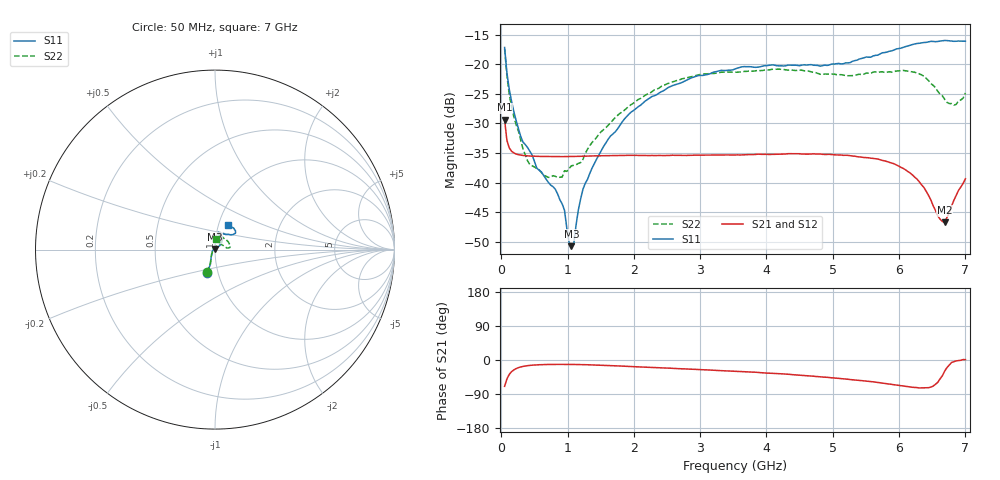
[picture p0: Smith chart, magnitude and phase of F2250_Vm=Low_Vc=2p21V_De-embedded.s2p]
! Integrated Device Technology
! Corporate Headquarters
! 6024 Silver Creek Valley Road
! San Jose, CA 95138  USA
! Phone:  1-408-284-8200
! Toll Free:  1-800-223-1366
! Webpage:  http://www.idt.com/
! Timing and RF Division
! 515 Groton Road, Suite 102
! Westford, MA 01886-6024
! Device:  F2250
! Description: Voltage Variable RF Attenuator
! Frequency:  50.0 -  6000.00 MHz
! Package:  3x3 mm Thin QFN Plastic Package: 16 pin
! Ports:  2 RF, 3 DC
!  Pin  1  = GND
!  Pin  2  = NC
!  Pin  3  = RF1  = Port 1
!  Pin  4  = NC
!  Pin  5  = GND
!  Pin  6  = GND
!  Pin  7  = GND
!  Pin  8  = GND
!  Pin  9  = NC
!  Pin 10  = RF2  = Port 2
!  Pin 11  = NC
!  Pin 12  = GND
!  Pin 13  = GND
!  Pin 14  = VCNTRL
!  Pin 15  = VDD
!  Pin 16  = VMODE
! Vcntrl:  2.210 Volts
! Vmode:  +0.000 Volts
! Vdd:  +3.30  Volts
! Current:  1.178 mA
! Data:  The device was measured on a the F2250 evaluation board which has
!  individual transmission lines to the RF pins.  Data was collected
!  using a calibrated network analyzer.  The evaluation board was
!  de-embedded using a TRL calibration technique.
!  The reference plane is the edge of the package pin.
! Misc:  SN 10
!  Action Tracker AT0258
! Date Measured:  2014-11-26
! Date:  2015-10-15  MJV
! Note:
!  Integrated Device Technology supplies this data as a sample of measured
!  data at the package pin for this product.  Your particular data for this
!  product may vary.
!  Data was taken at 25 degrees C.
!  Integrated Device Technology reserves the right to change this data at anytime.
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# GHz S dB R 50
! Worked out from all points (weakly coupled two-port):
!   201 points, 50 MHz to 7 GHz, reference 50 ohm
!   highest |S21| = -29.38 dB at 50 MHz (marker M1); lowest = -46.7 dB at 6.687 GHz (marker M2)
!   lowest |S11| = -50.7 dB at 1.058 GHz (marker M3), VSWR 1.01, Z = 49.8 + j0.245 ohm
!   |S11| at or under -10 dB: start of sweep to end of sweep
!   |S22| runs from -39.1 to -17.4 dB; largest |S21 - S12| = 6.7e-05
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0.05  -17.18 -108.6  -29.38 -69.5  -29.38 -69.5  -17.39 -110.5
0.08475  -21.44 -107.4  -32.86 -50.0  -32.86 -50.0  -21.92 -108.8
0.15425  -26.23 -116.6  -34.67 -30.9  -34.68 -30.9  -27.14 -119.9
0.29325  -32.20 -127.7  -35.34 -18.4  -35.34 -18.3  -32.79 -133.2
0.3975  -34.08 -141.7  -35.47 -15.0  -35.47 -14.9  -36.32 -156.9
0.71025  -39.96 -168.3  -35.58 -11.8  -35.59 -11.8  -39.10 153.4
0.91875  -43.59 158.3  -35.60 -11.5  -35.59 -11.6  -39.03 126.3
0.9535  -44.65 169.4  -35.59 -11.5  -35.59 -11.6  -37.98 124.6
1.023  -50.07 143.7  -35.59 -11.6  -35.58 -11.6  -37.60 107.6
1.05775  -50.71 122.4  -35.58 -11.7  -35.58 -11.7  -37.14 102.3
1.0925  -50.40 90.9  -35.57 -11.8  -35.57 -11.8  -37.05 97.4
1.162  -44.61 56.9  -35.55 -11.9  -35.55 -11.9  -36.74 86.2
1.2315  -41.10 44.0  -35.52 -12.2  -35.53 -12.2  -36.06 76.8
1.6485  -32.11 41.9  -35.44 -14.7  -35.43 -14.8  -29.87 60.0
2.37825  -24.87 47.3  -35.39 -20.4  -35.39 -20.4  -24.03 54.6
3.525  -20.80 72.5  -35.33 -29.7  -35.33 -29.7  -21.38 73.7
4.7065  -20.17 72.3  -35.13 -42.7  -35.14 -42.8  -21.38 71.7
5.85325  -17.82 40.5  -36.56 -63.4  -36.55 -63.5  -21.28 21.8
6.27025  -16.51 40.1  -39.39 -72.8  -39.39 -72.7  -21.48 8.5
6.68725  -15.99 48.8  -46.68 -29.4  -46.65 -28.9  -25.92 27.5
6.861  -16.12 55.1  -42.16 -2.4  -42.12 -2.5  -26.79 58.0
7  -16.12 63.2  -39.34 1.0  -39.30 0.8  -24.86 84.0
